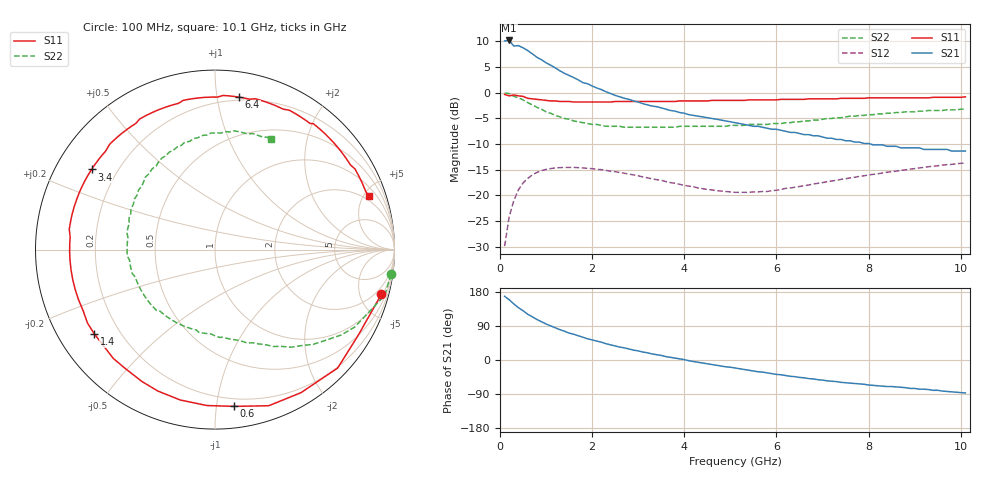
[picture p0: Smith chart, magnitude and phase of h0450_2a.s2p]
!HBFP-0450
!S and NOISE PARAMETERS at Vce=2V  Ic=1mA.  LAST UPDATED  09-04-98
# GHZ S MA R  50
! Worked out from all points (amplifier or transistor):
!   101 points, 100 MHz to 10.1 GHz, reference 50 ohm
!   highest |S21| = 10.2 dB at 200 MHz (marker M1)
!   |S21| within 3 dB of that: start of sweep to 760.4 MHz
!   unconditionally stable (mu >= 1): 3.319 GHz to end of sweep
!   at 1.7 GHz: K = 0.45, MSG = 8.5 dB, |S12| = -14.6 dB
!   at 5.1 GHz: K = 1.70, MAG = 1.9 dB, |S12| = -19.4 dB
!   at 10.1 GHz: K = 1.23, MAG = -1.7 dB, |S12| = -13.7 dB
!   lowest NFmin = 2.01 dB at 2 GHz
!   S11 on the Smith chart (normalised r, x): 100 MHz: 1.17, -7.41; 600 MHz: 0.14, -1.12; 1.4 GHz: 0.11, -0.31; 3.4 GHz: 0.11, +0.29; 6.4 GHz: 0.18, +1.16; 10.1 GHz: 1.60, +5.52
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0.1  0.96 -15.0  3.19 168.0  0.032 81.0  0.99 -8.0
0.2  0.93 -31.0  3.22 159.0  0.062 72.0  0.98 -15.0
0.3  0.95 -44.0  2.84 148.0  0.089 62.0  0.92 -23.0
0.4  0.93 -59.0  2.87 138.0  0.113 54.0  0.89 -29.0
0.6  0.88 -83.0  2.57 121.0  0.146 39.0  0.8 -39.0
0.8  0.86 -103.0  2.21 107.0  0.167 28.0  0.72 -48.0
1  0.84 -119.0  1.95 95.0  0.179 19.0  0.65 -56.0
1.2  0.83 -133.0  1.74 85.0  0.185 11.0  0.6 -62.0
1.4  0.82 -145.0  1.54 76.0  0.187 4.0  0.56 -68.0
1.5  0.82 -150.0  1.47 71.0  0.187 1.0  0.55 -71.0
1.8  0.81 -164.0  1.25 60.0  0.185 -7.0  0.51 -79.0
2.6  0.82 168.0  0.91 34.0  0.167 -22.0  0.47 -101.0
3.4  0.82 147.0  0.73 14.0  0.142 -32.0  0.46 -122.0
3.5  0.82 145.0  0.71 12.0  0.14 -33.0  0.46 -124.0
4.1  0.83 131.0  0.61 -2.0  0.123 -35.0  0.47 -140.0
5.1  0.84 109.0  0.51 -21.0  0.107 -32.0  0.48 -167.0
6.4  0.86 81.0  0.41 -44.0  0.12 -26.0  0.52 154.0
6.8  0.87 73.0  0.38 -50.0  0.129 -27.0  0.54 142.0
7.6  0.88 58.0  0.34 -61.0  0.148 -32.0  0.59 120.0
8.5  0.89 44.0  0.3 -70.0  0.17 -40.0  0.63 99.0
9.3  0.89 32.0  0.28 -78.0  0.19 -50.0  0.67 81.0
10.1  0.91 19.0  0.27 -87.0  0.206 -62.0  0.69 63.0
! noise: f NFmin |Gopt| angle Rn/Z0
1.8  2.05  0.66  150  0.12
2  2.01  0.69  160  0.08
2.5  2.37  0.73  180  0.05
3.5  2.81  0.79  -149  0.26
4  3.08  0.81  -136  0.57
5  3.52  0.85  -113  1.7
5.5  3.74  0.88  -101  2.66
7  4.43  0.9  -70  6.52
8  4.87  0.89  -53  9.46
10  5.78  0.84  -21  12.16
